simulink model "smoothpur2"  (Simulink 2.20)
settings: Solver=ode45  StartTime=0  StopTime=5.0  MaxStep=.01  RelTol=1e-3  AbsTol=1e-3
undefined symbols (not defined in the file or in its folder): sfuny

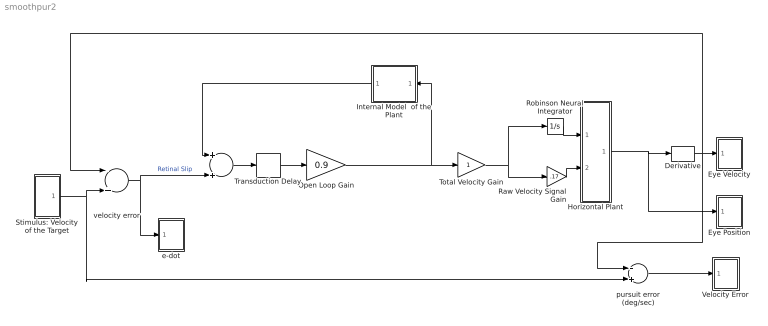
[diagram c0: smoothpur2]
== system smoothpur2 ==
  "  " : Sum  Inputs=++
  Derivative : Derivative
  Eye Position : Subsystem  LoadFcn=sfuny([],[],[],'LoadBlock')  StartFcn=sfuny([],[],[],'Start')  StopFcn=sfuny([],[],[],'Stop')  mask(Graph scope.){}
      mask help: Graph scope using MATLAB graph window. Enter plotting ranges and line type.
      mask init:
      | color = @4; ax = [0, @1, @2, @3]; dt = -1;
  Eye Velocity : Subsystem  LoadFcn=sfuny([],[],[],'LoadBlock')  StartFcn=sfuny([],[],[],'Start')  StopFcn=sfuny([],[],[],'Stop')  mask(Graph scope.){}
      mask help: Graph scope using MATLAB graph window. Enter plotting ranges and line type.
      mask init:
      | color = @4; ax = [0, @1, @2, @3]; dt = -1;
  Horizontal Plant : Subsystem
  Internal Model  of the Plant : Subsystem  Orientation=left
  Open Loop Gain : Gain  Gain=0.9
  Raw Velocity Signal Gain : Gain  Gain=.17
  Robinson Neural Integrator : Integrator  ExternalReset=none  InitialConditionSource=internal  InitialCondition=0  LimitOutput=off  UpperSaturationLimit=inf  LowerSaturationLimit=-inf  ShowSaturationPort=off  ShowStatePort=off  AbsoluteTolerance=auto
  Stimulus: Velocity of the Target : Subsystem
  Total Velocity Gain : Gain  Gain=1
  Transduction Delay : TransportDelay  DelayTime=.07  InitialInput=00  BufferSize=1024
  Velocity Error : Subsystem  LoadFcn=sfuny([],[],[],'LoadBlock')  StartFcn=sfuny([],[],[],'Start')  StopFcn=sfuny([],[],[],'Stop')  mask(Graph scope.){}
      mask help: Graph scope using MATLAB graph window. Enter plotting ranges and line type.
      mask init:
      | color = @4; ax = [0, @1, @2, @3]; dt = -1;
  e-dot : Subsystem  LoadFcn=sfuny([],[],[],'LoadBlock')  StartFcn=sfuny([],[],[],'Start')  StopFcn=sfuny([],[],[],'Stop')  mask(Graph scope.){}
      mask help: Graph scope using MATLAB graph window. Enter plotting ranges and line type.
      mask init:
      | color = @4; ax = [0, @1, @2, @3]; dt = -1;
  pursuit error (deg/sec) : Sum  Inputs=-+
  velocity error : Sum  Inputs=-+
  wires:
  Raw Velocity Signal Gain/1 -> Horizontal Plant/2(in_2)
  Robinson Neural Integrator/1 -> Horizontal Plant/1(in_1)
  Horizontal Plant/1(out_1) -> Derivative/1, Eye Position/1(x)
  Stimulus: Velocity of the Target/1(out_1) -> velocity error/2, pursuit error (deg/sec)/2
  pursuit error (deg/sec)/1 -> Velocity Error/1(x)
  Derivative/1 -> pursuit error (deg/sec)/1, Eye Velocity/1(x), velocity error/1
  Total Velocity Gain/1 -> Robinson Neural Integrator/1, Raw Velocity Signal Gain/1
  "  "/1 -> Transduction Delay/1
  Transduction Delay/1 -> Open Loop Gain/1
  velocity error/1 -> e-dot/1(x), "  "/2  "Retinal Slip"
  Open Loop Gain/1 -> Total Velocity Gain/1, Internal Model  of the Plant/1(In1)
  Internal Model  of the Plant/1(Out1) -> "  "/1

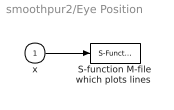
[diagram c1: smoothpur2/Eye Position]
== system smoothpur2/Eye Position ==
  x : Inport  Port=1  PortWidth=-1  SampleTime=-1
  "S-function M-file which plots lines " : S-Function  FunctionName=sfuny  Parameters=ax, color,dt  PortCounts=[]  SFunctionModules=''
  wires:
  x/1 -> "S-function M-file which plots lines "/1

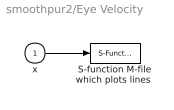
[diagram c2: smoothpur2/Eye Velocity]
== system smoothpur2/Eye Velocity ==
  x : Inport  Port=1  PortWidth=-1  SampleTime=-1
  "S-function M-file which plots lines " : S-Function  FunctionName=sfuny  Parameters=ax, color,dt  PortCounts=[]  SFunctionModules=''
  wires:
  x/1 -> "S-function M-file which plots lines "/1

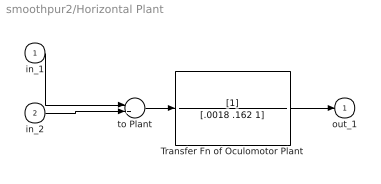
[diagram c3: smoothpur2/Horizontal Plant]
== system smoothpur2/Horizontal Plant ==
  in_1 : Inport  Port=1  PortWidth=-1  SampleTime=-1
  in_2 : Inport  Port=2  PortWidth=-1  SampleTime=-1
  Transfer Fn of Oculomotor Plant : TransferFcn  Numerator=[1]  Denominator=[.0018 .162 1]
  to Plant : Sum  Inputs=++
  out_1 : Outport  Port=1  InitialOutput=0
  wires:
  Transfer Fn of Oculomotor Plant/1 -> out_1/1
  in_2/1 -> to Plant/2
  in_1/1 -> to Plant/1
  to Plant/1 -> Transfer Fn of Oculomotor Plant/1

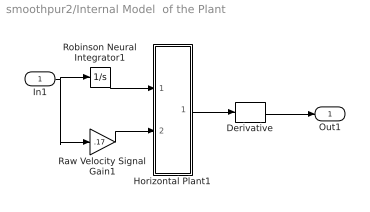
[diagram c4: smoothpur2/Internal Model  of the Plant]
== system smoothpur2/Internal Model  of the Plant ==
  In1 : Inport  Port=1  PortWidth=-1  SampleTime=-1
  Derivative : Derivative
  Horizontal Plant1 : Subsystem
  Raw Velocity Signal Gain1 : Gain  Gain=.17
  Robinson Neural Integrator1 : Integrator  ExternalReset=none  InitialConditionSource=internal  InitialCondition=0  LimitOutput=off  UpperSaturationLimit=inf  LowerSaturationLimit=-inf  ShowSaturationPort=off  ShowStatePort=off  AbsoluteTolerance=auto
  Out1 : Outport  Port=1  InitialOutput=0
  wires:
  Raw Velocity Signal Gain1/1 -> Horizontal Plant1/2(in_2)
  Robinson Neural Integrator1/1 -> Horizontal Plant1/1(in_1)
  In1/1 -> Robinson Neural Integrator1/1, Raw Velocity Signal Gain1/1
  Horizontal Plant1/1(out_1) -> Derivative/1
  Derivative/1 -> Out1/1

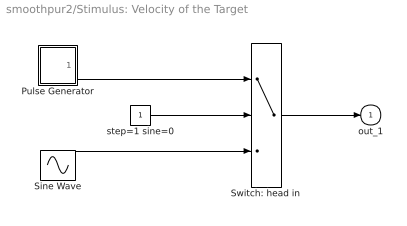
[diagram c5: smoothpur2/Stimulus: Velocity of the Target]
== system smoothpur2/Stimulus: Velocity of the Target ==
  Pulse Generator : Subsystem  mask(Pulse Generator){}
      mask help: Pulse Generator.
      mask init:
      | Ts=@1; du=@2; ht=@3; stt=@4; ini=ones(length(ht),1); st1=rem(stt,Ts); st2=rem(stt+du,Ts);if(Ts<=1.2*du),ini=zeros(length(ht),1);end;
  Sine Wave : Sin  Amplitude=10  Frequency=1*pi*2  Phase=0  SampleTime=-1
  Switch: head in : Switch  Threshold=.5
  step=1 sine=0 : Constant  Value=1
  out_1 : Outport  Port=1  InitialOutput=0
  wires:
  Sine Wave/1 -> Switch: head in/3
  Pulse Generator/1(out_1) -> Switch: head in/1
  Switch: head in/1 -> out_1/1
  step=1 sine=0/1 -> Switch: head in/2

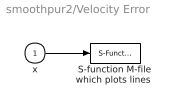
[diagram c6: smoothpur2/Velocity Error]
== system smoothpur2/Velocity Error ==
  x : Inport  Port=1  PortWidth=-1  SampleTime=-1
  "S-function M-file which plots lines " : S-Function  FunctionName=sfuny  Parameters=ax, color,dt  PortCounts=[]  SFunctionModules=''
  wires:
  x/1 -> "S-function M-file which plots lines "/1

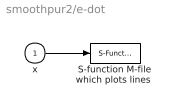
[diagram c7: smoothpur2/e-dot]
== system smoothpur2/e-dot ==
  x : Inport  Port=1  PortWidth=-1  SampleTime=-1
  "S-function M-file which plots lines " : S-Function  FunctionName=sfuny  Parameters=ax, color,dt  PortCounts=[]  SFunctionModules=''
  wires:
  x/1 -> "S-function M-file which plots lines "/1

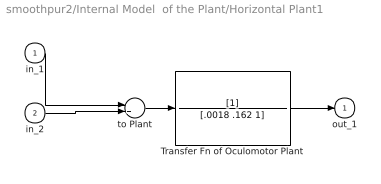
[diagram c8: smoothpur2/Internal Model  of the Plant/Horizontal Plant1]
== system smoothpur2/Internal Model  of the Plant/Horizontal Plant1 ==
  in_1 : Inport  Port=1  PortWidth=-1  SampleTime=-1
  in_2 : Inport  Port=2  PortWidth=-1  SampleTime=-1
  Transfer Fn of Oculomotor Plant : TransferFcn  Numerator=[1]  Denominator=[.0018 .162 1]
  to Plant : Sum  Inputs=++
  out_1 : Outport  Port=1  InitialOutput=0
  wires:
  Transfer Fn of Oculomotor Plant/1 -> out_1/1
  in_2/1 -> to Plant/2
  in_1/1 -> to Plant/1
  to Plant/1 -> Transfer Fn of Oculomotor Plant/1

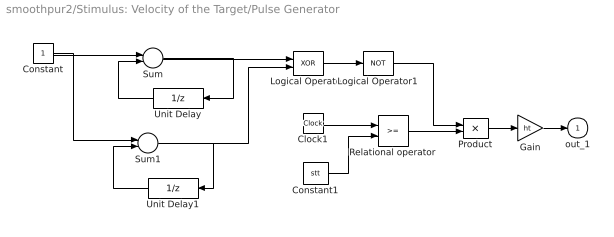
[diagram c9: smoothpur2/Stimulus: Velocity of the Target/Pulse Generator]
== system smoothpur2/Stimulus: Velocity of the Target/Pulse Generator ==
  Clock1 : Clock
  Constant : Constant  Value=1
  Constant1 : Constant  Value=stt
  Gain : Gain  Gain=ht
  Logical Operator : Logic  Operator=XOR  Inputs=2
  Logical Operator1 : Logic  Operator=NOT  Inputs=1
  Product : Product  Inputs=2
  Relational operator : RelationalOperator  Operator=>=
  Sum : Sum  Inputs=+-
  Sum1 : Sum  Inputs=+-
  Unit Delay : UnitDelay  Orientation=left  X0=0  SampleTime=[Ts,st1]
  Unit Delay1 : UnitDelay  Orientation=left  X0=ini  SampleTime=[Ts,st2]
  out_1 : Outport  Port=1  InitialOutput=0
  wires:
  Sum1/1 -> Logical Operator/2, Unit Delay1/1
  Sum/1 -> Logical Operator/1, Unit Delay/1
  Constant/1 -> Sum1/1, Sum/1
  Unit Delay1/1 -> Sum1/2
  Unit Delay/1 -> Sum/2
  Clock1/1 -> Relational operator/1
  Relational operator/1 -> Product/2
  Product/1 -> Gain/1
  Gain/1 -> out_1/1
  Constant1/1 -> Relational operator/2
  Logical Operator/1 -> Logical Operator1/1
  Logical Operator1/1 -> Product/1
